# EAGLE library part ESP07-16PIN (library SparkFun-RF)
Espressif ESP-07S WiFi-compatible SoC microcontroller. 16 GPIO pins User Guide
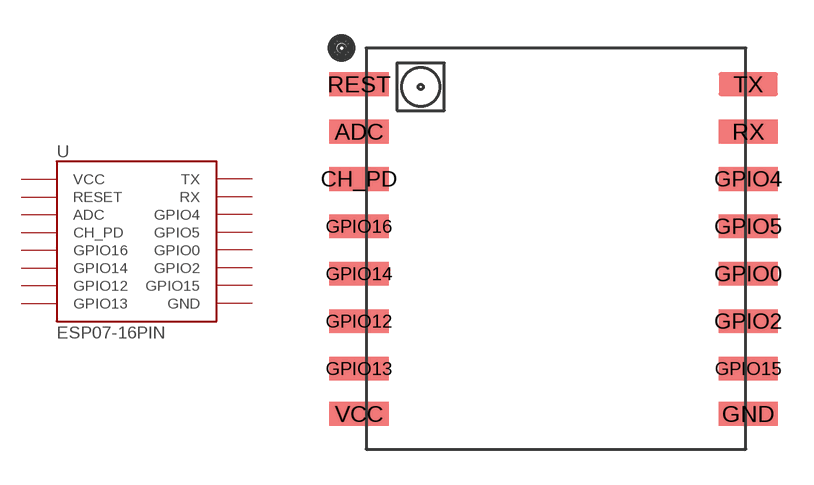
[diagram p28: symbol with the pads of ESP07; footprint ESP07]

Designator prefix -

## ESP07-16PIN (PROD_ID: IC-13915)  [ESP07]
ADC  ADC
CH_PD  CH_PD
GND  GND
GPIO0  GPIO0
GPIO2  GPIO2
GPIO4  GPIO4
GPIO5  GPIO5
GPIO12  GPIO12
GPIO13  GPIO13
GPIO14  GPIO14
GPIO15  GPIO15
GPIO16  GPIO16
REST  RESET
RX  RX
TX  TX
VCC  VCC

## Footprint ESP07 (pad centres in mm)
smd 2.5 x 1: ADC -8.026,3.841; CH_PD -8.026,1.841; GND 8.374,-8.064; GPIO0 8.374,-2.159; GPIO2 8.374,-4.159; GPIO4 8.374,1.841; GPIO5 8.374,-0.159; GPIO12 -8.026,-4.159; GPIO13 -8.026,-6.159; GPIO14 -8.026,-2.159; GPIO15 8.374,-6.159; GPIO16 -8.026,-0.159; REST -8.026,5.841; RX 8.374,3.841; TX 8.374,5.841; VCC -8.026,-8.064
